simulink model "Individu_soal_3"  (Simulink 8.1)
settings: Solver=ode45  StartTime=0.0  StopTime=5  RelTol=1e-3

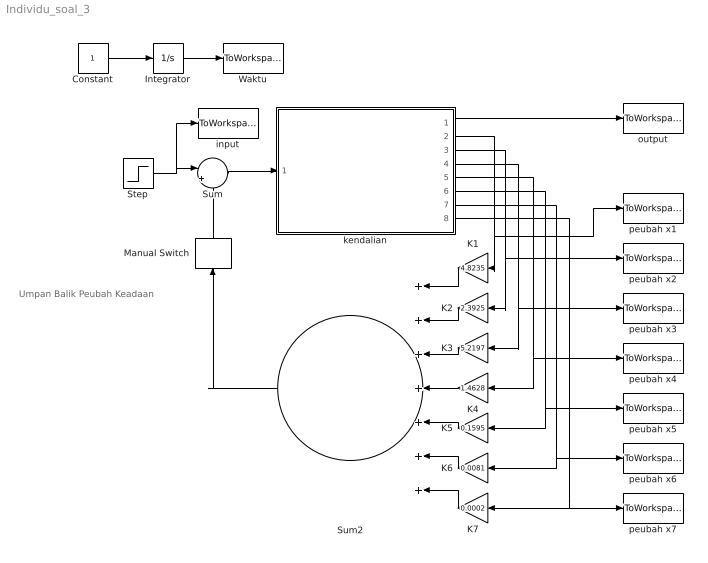
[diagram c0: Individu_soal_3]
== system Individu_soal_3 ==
  note: Umpan Balik Peubah Keadaan
  Constant : Constant
  Integrator : Integrator
  K1 : Gain  Gain=4.8235
  K2 : Gain  Gain=2.3925
  K3 : Gain  Gain=5.2197
  K4 : Gain  Gain=1.4628
  K5 : Gain  Gain=0.1595
  K6 : Gain  Gain=0.0081
  K7 : Gain  Gain=0.0002
  Manual Switch : ManualSwitch
  Step : Step  SampleTime=0
  Sum : Sum  Inputs=|+-
  Sum2 : Sum  Inputs=+++++++
  Waktu : ToWorkspace  VariableName=time  SampleTime=-1
  input : ToWorkspace  VariableName=u  SampleTime=-1
  kendalian : Subsystem
  output : ToWorkspace  VariableName=y  SampleTime=-1
  peubah x1 : ToWorkspace  VariableName=x1  SampleTime=-1
  peubah x2 : ToWorkspace  VariableName=x2  SampleTime=-1
  peubah x3 : ToWorkspace  VariableName=x3  SampleTime=-1
  peubah x4 : ToWorkspace  VariableName=x4  SampleTime=-1
  peubah x5 : ToWorkspace  VariableName=x5  SampleTime=-1
  peubah x6 : ToWorkspace  VariableName=x6  SampleTime=-1
  peubah x7 : ToWorkspace  VariableName=x7  SampleTime=-1
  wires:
  Constant/1 -> Integrator/1
  Integrator/1 -> Waktu/1
  kendalian/1(y) -> output/1
  Step/1 -> Sum/1, input/1
  kendalian/3(x2) -> K2/1, peubah x2/1
  K1/1 -> Sum2/1
  K2/1 -> Sum2/2
  Sum/1 -> kendalian/1(u)
  Sum2/1 -> Manual Switch/1
  Manual Switch/1 -> Sum/2
  kendalian/2(x1) -> K1/1, peubah x1/1
  K3/1 -> Sum2/3
  K4/1 -> Sum2/4
  kendalian/4(x3) -> K3/1, peubah x3/1
  K5/1 -> Sum2/5
  K6/1 -> Sum2/6
  kendalian/7(x6) -> K6/1, peubah x6/1
  K7/1 -> Sum2/7
  kendalian/5(x4) -> K4/1, peubah x4/1
  kendalian/6(x5) -> K5/1, peubah x5/1
  kendalian/8(x7) -> K7/1, peubah x7/1

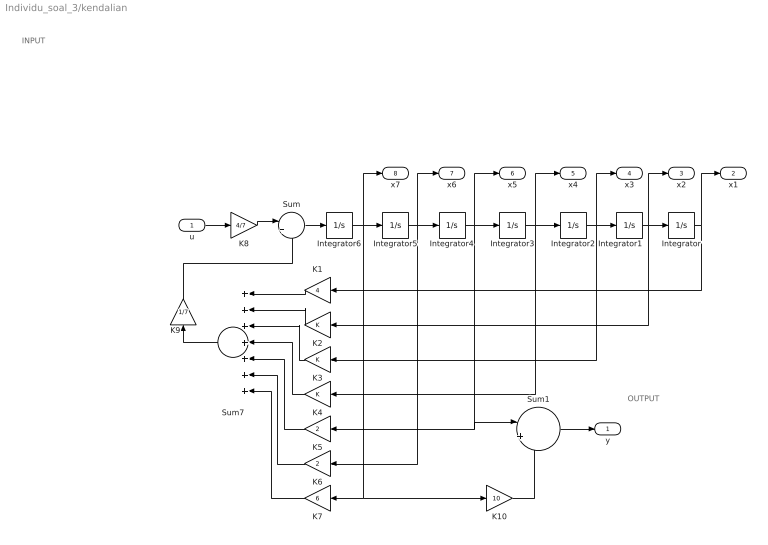
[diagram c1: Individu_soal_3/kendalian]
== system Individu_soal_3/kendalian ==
  note: INPUT
  note: OUTPUT
  u : Inport
  Integrator{,1..6} (7 alike) : Integrator
  K1 : Gain  Gain=4
  K10 : Gain  Gain=10
  K2 : Gain
  K3 : Gain
  K4 : Gain
  K5 : Gain  Gain=2
  K6 : Gain  Gain=2
  K7 : Gain  Gain=6
  K8 : Gain  Gain=4/7
  K9 : Gain  Gain=1/7
  Sum : Sum  Inputs=|++
  Sum1 : Sum  Inputs=|++
  Sum7 : Sum  Inputs=+++++++
  y : Outport
  x1 : Outport  Port=2
  x2 : Outport  Port=3
  x3 : Outport  Port=4
  x4 : Outport  Port=5
  x5 : Outport  Port=6
  x6 : Outport  Port=7
  x7 : Outport  Port=8
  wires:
  Sum1/1 -> y/1
  Integrator5/1 -> x6/1, K6/1, Integrator4/1
  u/1 -> K8/1
  K1/1 -> Sum7/1
  K2/1 -> Sum7/2
  K3/1 -> Sum7/3
  K4/1 -> Sum7/4
  K5/1 -> Sum7/5
  K6/1 -> Sum7/6
  K7/1 -> Sum7/7
  Sum7/1 -> K9/1
  Sum/1 -> Integrator6/1
  K9/1 -> Sum/2
  K8/1 -> Sum/1
  K10/1 -> Sum1/2
  Integrator6/1 -> x7/1, K10/1, K7/1, Integrator5/1
  Integrator3/1 -> x4/1, K4/1, Integrator2/1
  Integrator2/1 -> x3/1, K3/1, Integrator1/1
  Integrator/1 -> K1/1, x1/1
  Integrator1/1 -> x2/1, K2/1, Integrator/1
  Integrator4/1 -> x5/1, Sum1/1, K5/1, Integrator3/1
